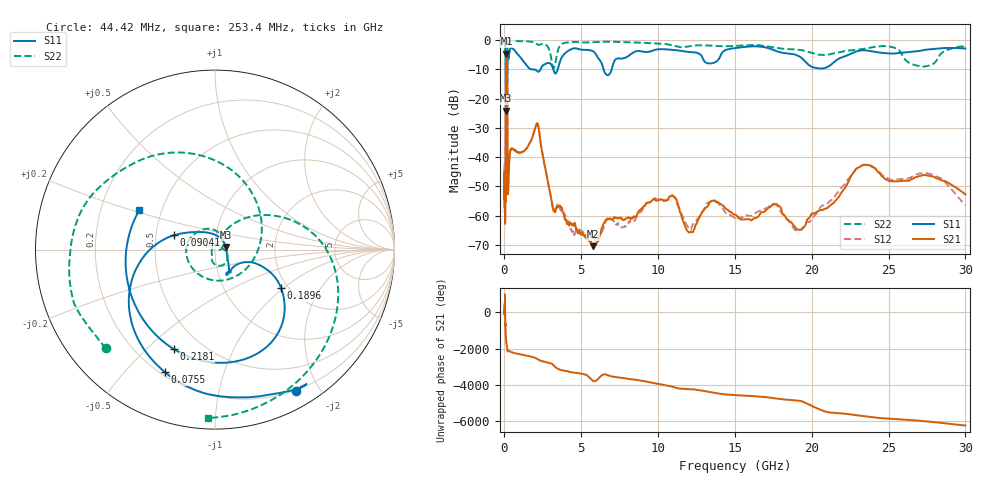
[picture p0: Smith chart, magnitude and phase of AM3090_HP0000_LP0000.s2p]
! Date/Time: Thu, Feb 28, 2019 1:52 PM
! Network Analyzer: Agilent Technologies E8364B Rev: A.07.50.67
! Sweep from 0.010 to 30.000 GHz, 1601 Points, Sweep Type: LOG
! Power Supply: 5.023 V, 0.002 A
# Hz S DB R 50
!freq MagS11 AngS11 MagS21 AngS21 MagS12 AngS12 MagS22 AngS22
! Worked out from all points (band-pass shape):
!   1601 points, 10 MHz to 30 GHz, reference 50 ohm
!   highest |S21| = -4.69 dB at 132.9 MHz (marker M1); lowest = -70.5 dB at 5.783 GHz (marker M2)
!   |S21| within 3 dB of the highest: 97.66 MHz to 174 MHz (76.35 MHz wide, 56.2 % of centre)
!   lowest |S11| = -24.1 dB at 97.94 MHz (marker M3), VSWR 1.13, Z = 56.4 + j1.58 ohm
!   |S11| at or under -10 dB: 1.785 GHz to 2.351 GHz (565.9 MHz wide, 27.4 % of centre); 3.18 GHz to 3.465 GHz (285 MHz wide, 8.58 % of centre); 6.454 GHz to 6.98 GHz (525.5 MHz wide, 7.82 % of centre)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
!   |S22| runs from -36.0 to -0.1 dB; largest |S21 - S12| = 0.012
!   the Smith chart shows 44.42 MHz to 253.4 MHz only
!   S11 on the Smith chart (normalised r, x): 44.42 MHz: 0.19, -1.71; 75.5 MHz: 0.22, -0.65; 90.41 MHz: 0.62, +0.10; 189.6 MHz: 1.84, -0.97; 218.1 MHz: 0.35, -0.61; 253.4 MHz: 0.37, +0.21
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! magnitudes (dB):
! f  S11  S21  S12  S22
! 10 MHz  -0.3  -45.6  -44.4  -0.5
! 38.04 MHz  -0.5  -60.4  -59.7  -1.3
! 44.42 MHz  -0.8  -58.6  -57.3  -1.7
! 69.7 MHz  -2.0  -53.8  -52.0  -3.6
! 75.5 MHz  -2.6  -42.4  -43.7  -5.1
! 90.41 MHz  -12.3  -13.5  -13.5  -15.4
! 97.94 MHz  -24.1  -7.6  -7.6  -16.4
! 132.9 MHz  -16.7  -4.7  -4.7  -30.9
! 144.7 MHz  -16.2  -4.9  -4.8  -21.1
! 169.8 MHz  -15.1  -6.8  -6.8  -35.9
! 189.6 MHz  -7.4  -19.2  -19.1  -9.9
! 218.1 MHz  -4.4  -52.1  -51.9  -1.5
! 253.4 MHz  -6.5  -49.9  -50.1  -0.5
! 550.5 MHz  -3.0  -37.2  -37.1  -0.2
! 2.084 GHz  -10.5  -28.7  -28.8  -1.3
! 3.188 GHz  -10.1  -58.3  -57.6  -9.6
! 5.783 GHz  -3.8  -70.5  -68.4  -0.7
! 7.926 GHz  -5.9  -61.0  -63.7  -0.7
! 10.7 GHz  -3.3  -53.8  -54.3  -1.6
! 19.31 GHz  -6.0  -64.9  -65.0  -3.4
! 23.48 GHz  -3.5  -42.7  -42.6  -2.9
! 30 GHz  -2.9  -52.8  -56.4  -2.2
